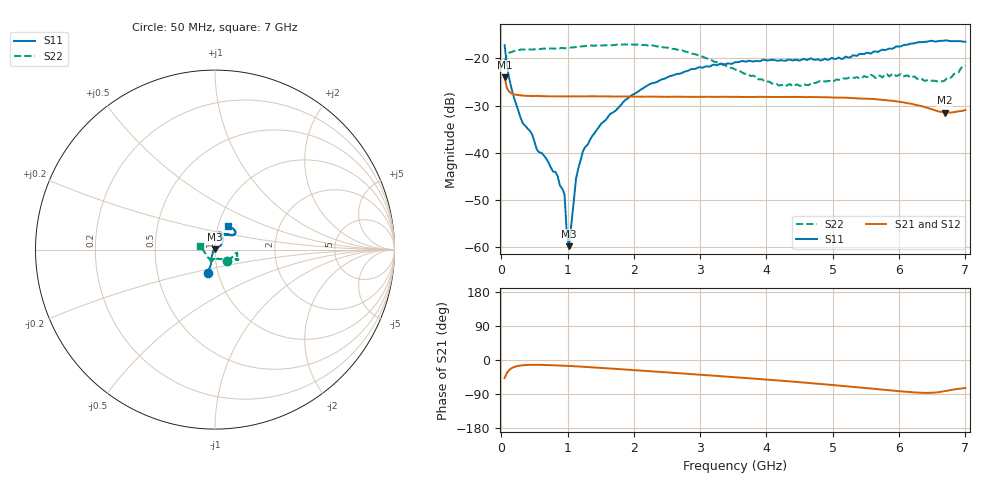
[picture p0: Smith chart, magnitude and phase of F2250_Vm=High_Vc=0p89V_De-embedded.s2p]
! Integrated Device Technology
! Corporate Headquarters
! 6024 Silver Creek Valley Road
! San Jose, CA 95138  USA
! Phone:  1-408-284-8200
! Toll Free:  1-800-223-1366
! Webpage:  http://www.idt.com/
! Timing and RF Division
! 515 Groton Road, Suite 102
! Westford, MA 01886-6024
! Device:  F2250
! Description: Voltage Variable RF Attenuator
! Frequency:  50.0 -  6000.00 MHz
! Package:  3x3 mm Thin QFN Plastic Package: 16 pin
! Ports:  2 RF, 3 DC
!  Pin  1  = GND
!  Pin  2  = NC
!  Pin  3  = RF1  = Port 1
!  Pin  4  = NC
!  Pin  5  = GND
!  Pin  6  = GND
!  Pin  7  = GND
!  Pin  8  = GND
!  Pin  9  = NC
!  Pin 10  = RF2  = Port 2
!  Pin 11  = NC
!  Pin 12  = GND
!  Pin 13  = GND
!  Pin 14  = VCNTRL
!  Pin 15  = VDD
!  Pin 16  = VMODE
! Vcntrl:  0.890 Volts
! Vmode:  +3.300 Volts
! Vdd:  +3.30  Volts
! Current:  1.313 mA
! Data:  The device was measured on a the F2250 evaluation board which has
!  individual transmission lines to the RF pins.  Data was collected
!  using a calibrated network analyzer.  The evaluation board was
!  de-embedded using a TRL calibration technique.
!  The reference plane is the edge of the package pin.
! Misc:  SN 10
!  Action Tracker AT0258
! Date Measured:  2014-11-26
! Date:  2015-10-15  MJV
! Note:
!  Integrated Device Technology supplies this data as a sample of measured
!  data at the package pin for this product.  Your particular data for this
!  product may vary.
!  Data was taken at 25 degrees C.
!  Integrated Device Technology reserves the right to change this data at anytime.
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# GHz S dB R 50
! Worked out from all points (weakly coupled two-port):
!   201 points, 50 MHz to 7 GHz, reference 50 ohm
!   highest |S21| = -24.03 dB at 50 MHz (marker M1); lowest = -31.5 dB at 6.687 GHz (marker M2)
!   lowest |S11| = -59.8 dB at 1.023 GHz (marker M3), VSWR 1.00, Z = 50 + j0.101 ohm
!   |S11| at or under -10 dB: start of sweep to end of sweep
!   |S22| runs from -25.9 to -17.0 dB; largest |S21 - S12| = 0.00013
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0.05  -17.17 -107.0  -24.03 -47.6  -24.03 -47.6  -20.81 -42.2
0.08475  -21.50 -105.5  -26.28 -34.0  -26.27 -34.0  -19.13 -18.9
0.1195  -24.27 -109.5  -27.06 -26.3  -27.04 -26.2  -18.77 -12.5
0.29325  -32.70 -121.7  -27.84 -14.5  -27.85 -14.5  -18.12 -9.0
0.467  -36.18 -139.3  -27.97 -12.7  -27.95 -12.7  -18.12 -8.8
0.5365  -39.33 -146.3  -27.95 -12.7  -27.97 -12.7  -18.02 -10.0
0.8145  -44.06 172.7  -28.03 -14.1  -28.04 -14.1  -17.92 -13.9
0.9535  -48.79 178.0  -28.03 -15.1  -28.04 -15.1  -17.85 -16.0
0.98825  -57.29 173.5  -28.04 -15.4  -28.04 -15.4  -17.80 -16.4
1.023  -59.81 80.5  -28.05 -15.7  -28.04 -15.7  -17.71 -16.5
1.12725  -45.46 33.4  -28.05 -16.7  -28.05 -16.7  -17.57 -17.8
1.2315  -39.67 28.0  -28.03 -17.8  -28.04 -17.8  -17.41 -19.4
1.5095  -33.78 33.9  -28.04 -21.0  -28.05 -21.0  -17.26 -21.0
1.857  -28.97 35.5  -28.07 -25.0  -28.04 -25.0  -17.02 -23.2
2.37825  -24.74 44.2  -28.12 -31.2  -28.12 -31.2  -17.41 -25.2
2.86475  -22.25 55.5  -28.14 -37.1  -28.14 -37.1  -18.94 -27.9
3.525  -20.81 70.6  -28.16 -45.4  -28.14 -45.5  -22.32 -45.0
4.18525  -20.47 76.6  -28.16 -54.0  -28.16 -54.1  -25.74 -75.3
4.7065  -20.25 71.3  -28.19 -61.7  -28.19 -61.7  -25.17 -99.0
5.85325  -17.90 39.9  -28.94 -79.9  -28.93 -80.0  -23.82 -107.2
6.68725  -16.20 47.3  -31.52 -82.3  -31.51 -82.4  -24.69 -164.2
7  -16.46 61.9  -30.93 -73.9  -30.94 -74.1  -21.43 167.8
